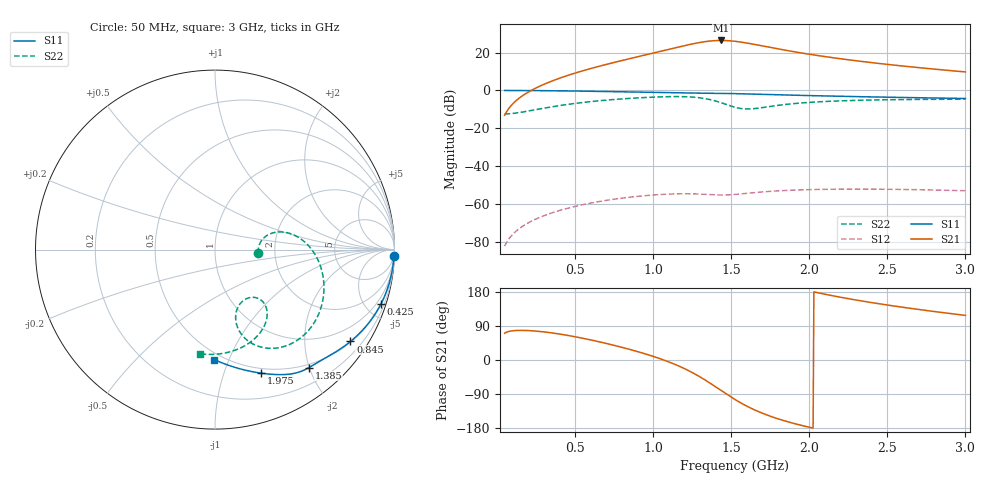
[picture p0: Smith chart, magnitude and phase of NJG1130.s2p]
! Created Thu May 17 19:20:05 2007
# hz S ma R 50
! 2 Port Network Data from SP1.SP block
! freq  magS11  angS11  magS21  angS21  magS12  angS12  magS22  angS22
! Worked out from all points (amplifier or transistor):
!   591 points, 50 MHz to 3 GHz, reference 50 ohm
!   highest |S21| = 26.4 dB at 1.435 GHz (marker M1)
!   |S21| within 3 dB of that: 1.187 GHz to 1.709 GHz (521.7 MHz wide, 36 % of centre)
!   unconditionally stable (mu >= 1): start of sweep to end of sweep
!   at 540 MHz: K = 10.66, MAG = 22.0 dB, |S12| = -60.5 dB
!   at 1.525 GHz: K = 3.89, MAG = 31.6 dB, |S12| = -54.9 dB
!   at 3 GHz: K = 29.27, MAG = 13.7 dB, |S12| = -52.9 dB
!   lowest NFmin = 0.39 dB at 990 MHz
!   S11 on the Smith chart (normalised r, x): 50 MHz: 4, -53; 425 MHz: 0.55, -6.27; 845 MHz: 0.52, -3.18; 1.385 GHz: 0.45, -2.00; 1.975 GHz: 0.45, -1.34; 3 GHz: 0.45, -0.89
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5e7  0.9972 -2.2  0.2203 70.6  7.77e-05 88.0  0.2401 -4.6
4.25e8  0.9731 -18.0  2.269 67.0  0.0007236 85.2  0.4116 13.3
5.45e8  0.9583 -22.8  3.251 57.8  0.0009561 81.7  0.4781 7.5
7e8  0.9356 -28.9  4.85 43.8  0.001254 75.9  0.5545 -2.2
8.45e8  0.9119 -34.2  6.809 28.7  0.001512 69.8  0.6148 -12.8
9.45e8  0.895 -37.6  8.54 16.9  0.001667 65.2  0.6494 -20.9
1.035e9  0.8801 -40.6  10.47 4.9  0.00178 60.9  0.6739 -29.0
1.145e9  0.8635 -44.0  13.44 -12.3  0.001867 55.5  0.6885 -40.3
1.25e9  0.8511 -47.1  16.82 -32.8  0.001871 50.8  0.6687 -52.9
1.32e9  0.8453 -49.3  19.02 -49.3  0.001823 48.8  0.6218 -62.1
1.385e9  0.8406 -51.4  20.45 -66.5  0.001764 49.0  0.5473 -69.6
1.435e9  0.836 -53.2  20.83 -80.3  0.00174 50.4  0.4755 -73.3
1.48e9  0.8304 -54.8  20.56 -92.6  0.001753 52.3  0.4115 -73.6
1.525e9  0.8232 -56.5  19.79 -104.2  0.001799 53.9  0.3604 -70.5
1.6e9  0.8086 -59.1  17.84 -121.6  0.001923 55.1  0.3244 -60.0
1.685e9  0.7905 -61.8  15.39 -137.9  0.002075 54.2  0.3454 -50.5
1.82e9  0.7631 -65.6  12.08 -157.8  0.002264 50.5  0.4135 -47.8
1.975e9  0.7351 -69.5  9.373 -175.0  0.002397 45.3  0.4759 -52.6
2.02e9  0.7277 -70.6  8.761 -179.3  0.002423 43.8  0.4898 -54.4
2.23e9  0.6963 -75.3  6.602 163.3  0.002487 36.5  0.536 -63.9
2.51e9  0.6612 -81.1  4.816 144.5  0.002466 26.2  0.5684 -76.7
3e9  0.6137 -90.3  3.076 117.7  0.002253 2.2  0.5867 -98.4
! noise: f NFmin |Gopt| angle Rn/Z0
5e+07  7.518  0.9961  2.161  694.8
3.75e+08  0.7703  0.947  15.81  2.605
7.05e+08  0.4397  0.8722  27.7  0.6002
1.03e+09  0.3894  0.8164  38.6  0.3708
1.36e+09  0.4413  0.7753  50.15  0.3186
1.685e+09  0.5604  0.7398  61.58  0.3016
2.015e+09  0.7553  0.704  72.65  0.2959
2.34e+09  1.035  0.6673  82.61  0.2978
2.67e+09  1.42  0.6287  91.54  0.3082
3e+09  1.912  0.5908  99.18  0.3293
